DATA_BLOCK "Data_1"
STRUCT
	VAR0		: INT
END_STRUCT
BEGIN
	VAR0		:= 123
END_DATA_BLOCK


ORGANIZATION_BLOCK OB 1
BEGIN
	// Test symbolic M access
	__STWRST
	U		"sym_M_0.0"
	__ASSERT==	__STW VKE,	0
	SET
	=		M 0.0
	__STWRST
	U		"sym_M_0.0"
	__ASSERT==	__STW VKE,	1
	CLR
	=		"sym_M_0.0"
	__STWRST
	U		M 0.0
	__ASSERT==	__STW VKE,	0


	// Test symbolic fully qualified access
	L		"Data_1".VAR0
	__ASSERT==	__ACCU 1,	123

END_ORGANIZATION_BLOCK
